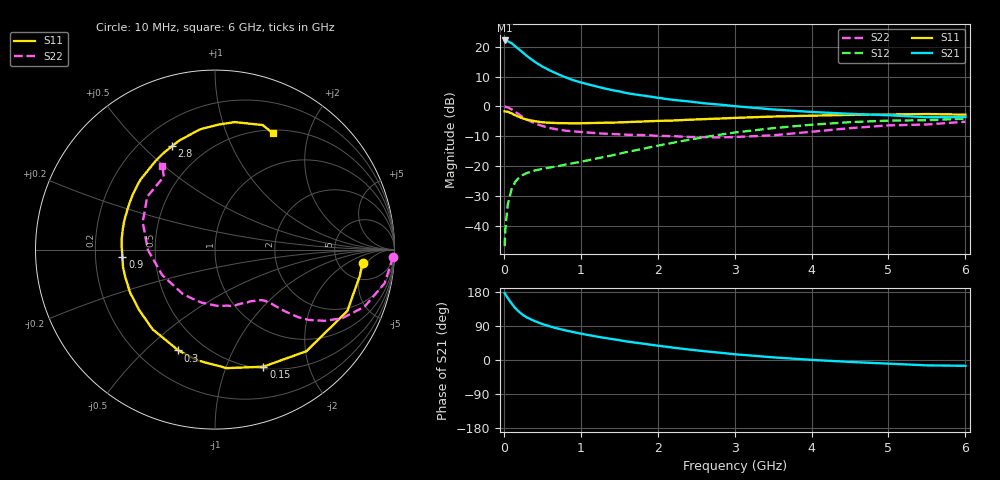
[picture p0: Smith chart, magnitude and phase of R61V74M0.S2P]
! SIEMENS Small Signal Semiconductors
! BFR193
! Si NPN RF Bipolar Junction Transistor in SOT23
! VCE = 1.75 V  IC = 4 mA
! Common Emitter S-Parameters:  May  1996
# GHz  S  MA  R  50
!  f  S11  S21  S12  S22
! GHz  MAG  ANG  MAG  ANG  MAG  ANG  MAG  ANG
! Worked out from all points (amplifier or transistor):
!   36 points, 10 MHz to 6 GHz, reference 50 ohm
!   highest |S21| = 22.1 dB at 10 MHz (marker M1)
!   |S21| within 3 dB of that: start of sweep to 197.6 MHz
!   unconditionally stable (mu >= 1): 946.7 MHz to 2.023 GHz
!   at 250 MHz: K = 0.37, MSG = 20.5 dB, |S12| = -23.0 dB
!   at 1.4 GHz: K = 1.08, MAG = 9.3 dB, |S12| = -16.5 dB
!   at 6 GHz: K = 0.98, MSG = 0.3 dB, |S12| = -4.1 dB
!   S11 on the Smith chart (normalised r, x): 10 MHz: 8.66, -3.91; 150 MHz: 0.52, -1.36; 300 MHz: 0.36, -0.64; 900 MHz: 0.32, -0.04; 2.8 GHz: 0.33, +0.62; 6 GHz: 0.54, +1.47
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0.01  0.8253 -5.0  12.76 177.0  0.0045 85.8  0.9935 -2.3
0.02  0.8197 -10.3  12.64 173.3  0.0088 83.3  0.9832 -4.6
0.05  0.8128 -24.9  12.34 163.9  0.0221 77.0  0.9636 -11.2
0.1  0.7614 -48.0  11.52 149.2  0.0409 66.8  0.8917 -20.9
0.15  0.706 -67.5  10.11 136.5  0.0546 58.5  0.805 -28.4
0.2  0.6637 -84.3  8.981 126.8  0.0643 52.5  0.7267 -33.1
0.25  0.625 -99.0  7.925 118.5  0.0711 48.1  0.6541 -36.8
0.3  0.5977 -110.0  6.994 112.2  0.0761 46.1  0.5976 -39.1
0.4  0.5639 -128.1  5.613 102.8  0.0836 43.2  0.521 -41.4
0.5  0.5402 -141.6  4.648 94.9  0.0894 42.6  0.4682 -42.8
0.6  0.5303 -153.1  3.993 88.5  0.0942 43.5  0.4318 -43.9
0.7  0.5232 -161.7  3.486 83.0  0.0989 44.7  0.4084 -45.1
0.9  0.5177 -175.4  2.758 73.8  0.1113 47.8  0.3802 -47.7
1.1  0.5237 172.7  2.332 65.8  0.1247 51.3  0.3633 -51.7
1.3  0.5302 162.9  2.009 58.7  0.1415 54.1  0.3478 -56.1
1.6  0.5436 150.6  1.667 48.9  0.1709 56.9  0.3338 -64.5
2.2  0.5781 130.3  1.284 32.6  0.2452 56.6  0.3164 -85.7
2.8  0.6236 112.7  1.072 19.4  0.3326 50.5  0.301 -114.8
3.5  0.6749 97.2  0.887 7.0  0.4308 39.4  0.3268 -154.3
4.5  0.719 81.1  0.749 -5.1  0.5428 21.8  0.4305 159.2
5.5  0.7431 69.1  0.657 -14.2  0.5851 4.5  0.4963 125.1
6  0.7244 63.7  0.662 -15.3  0.621 -0.4  0.5519 122.1
